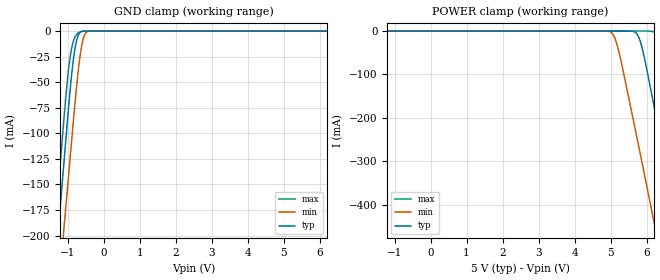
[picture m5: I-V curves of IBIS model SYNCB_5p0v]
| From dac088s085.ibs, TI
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|   Model
[Model]   SYNCB_5p0v
Model_type   Input
Vinl = 0.8
Vinh = 2.4
|   typ   min   max
C_comp   0.660pF   0.639pF   0.767pF
[Voltage Range]   5   4.5   5.5
[Temperature Range]   27   125   -40
[Power Clamp Reference]   5   4.5   5.5
[GND Clamp Reference]   0   0   0
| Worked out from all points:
|   GND clamp passes 1 mA (typ) near -0.64 V on its own axis
[GND Clamp]
|   Voltage   I(typ)   I(min)   I(max)
-5V       -1.813A    -1.827A    -1.812A
-1.355V   -235.3mA   -295.2mA   -195.6mA
-1.325V   -222.5mA   -282.9mA   -182.5mA
-1.235V   -184.3mA   -246.3mA   -143.1mA
-1.115V   -133.7mA   -197.8mA   -90.75mA
-995mV    -83.26mA   -149.6mA   -43.85mA
-905mV    -48.31mA   -113.7mA   -19.81mA
-785mV    -14.76mA   -66.35mA   -4.887mA
-635mV    -791uA     -19.45mA   -496.3uA
-515mV    -40.35uA   -2.742mA   -21.44uA
-365mV    -522.7nA   -51.88uA   0A
9.985V    0A         0A         0A
[POWER Clamp]
|   Voltage   I(typ)   I(min)   I(max)
-5V       0A         0A         0A
5.005V    0A         -2.188mA   0A
5.095V    0A         -11.61mA   0A
5.215V    0A         -41.65mA   0A
5.755V    -9.682mA   -254.4mA   0A
5.905V    -48.32mA   -315.6mA   -469.1nA
6.205V    -171.6mA   -439.3mA   -1.751mA
6.265V    -197mA     -464.2mA   -3.842mA
6.475V    -286.4mA   -551.6mA   -37.4mA
6.865V    -453.8mA   -714.9mA   -200mA
7.495V    -725.9mA   -979.8mA   -477.9mA
9.985V    -1.807A    -2.032A    -1.583A
